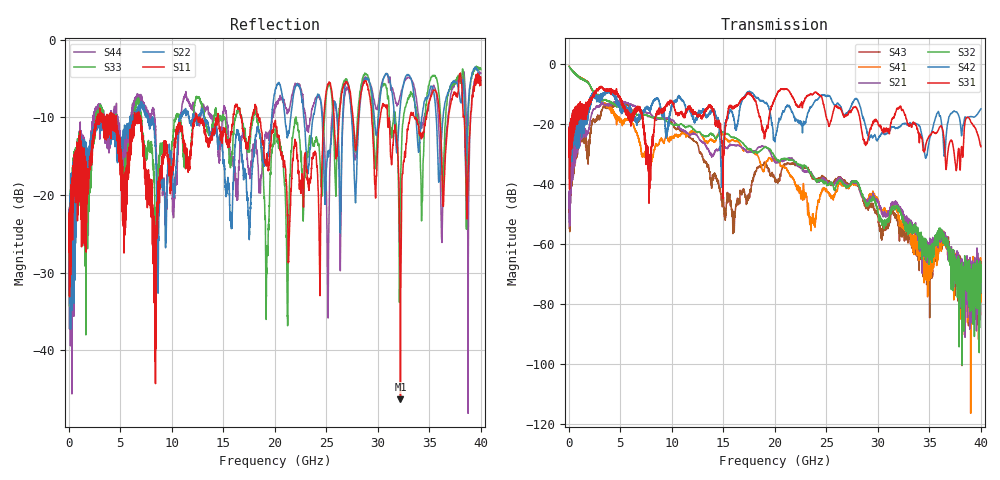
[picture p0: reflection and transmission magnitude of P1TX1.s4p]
!Agilent Technologies,N5245A,MY49151084,A.09.20.08
!Agilent N5245A: A.09.20.08
!Date: Thursday, March 01, 2012 10:29:25
!Correction: S11(Full 4 Port(1,2,3,4))
!S12(Full 4 Port(1,2,3,4))
!S13(Full 4 Port(1,2,3,4))
!S14(Full 4 Port(1,2,3,4))
!S21(Full 4 Port(1,2,3,4))
!S22(Full 4 Port(1,2,3,4))
!S23(Full 4 Port(1,2,3,4))
!S24(Full 4 Port(1,2,3,4))
!S31(Full 4 Port(1,2,3,4))
!S32(Full 4 Port(1,2,3,4))
!S33(Full 4 Port(1,2,3,4))
!S34(Full 4 Port(1,2,3,4))
!S41(Full 4 Port(1,2,3,4))
!S42(Full 4 Port(1,2,3,4))
!S43(Full 4 Port(1,2,3,4))
!S44(Full 4 Port(1,2,3,4))
!S4P File: Measurements: <S11,S12,S13,S14>,
!<S21,S22,S23,S24>,
!<S31,S32,S33,S34>,
!<S41,S42,S43,S44>:
# Hz S  dB  R 50
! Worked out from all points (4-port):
!   3996 points, 50 MHz to 40 GHz, reference 50 ohm
!   strongest paths, dB at 50 MHz, 10.04 GHz, 20.03 GHz, 30.02 GHz, 40 GHz:
!     S31: -23.6, -13.0, -11.5, -19.8, -27.5
!     S42: -23.5, -13.7, -25.9, -25.1, -15.0
!     S32: -0.8, -20.0, -31.2, -49.2, -67.6
!     S21: -43.5, -18.7, -32.8, -45.4, -76.0
!     S41: -0.7, -24.3, -31.7, -45.5, -64.7
!     S43: -44.3, -19.7, -38.9, -50.6, -71.4
!   lowest |S11| = -46.4 dB at 32.2 GHz (marker M1), VSWR 1.01, Z = 50.2 + j0.429 ohm
!   |S11| at or under -10 dB: start of sweep to 2.749 GHz; 6.99 GHz to 12.31 GHz (5.318 GHz wide, 55.1 % of centre); 18.41 GHz to 24.76 GHz (6.352 GHz wide, 29.4 % of centre)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
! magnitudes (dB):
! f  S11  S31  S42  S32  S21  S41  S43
! 50 MHz  -23.4  -23.6  -23.5  -0.8  -43.5  -0.7  -44.3
! 5.4 GHz  -22.8  -15.0  -13.9  -15.1  -12.7  -19.1  -13.0
! 7.79 GHz  -18.6  -38.8  -15.2  -17.3  -16.2  -36.9  -17.4
! 15.98 GHz  -9.7  -14.7  -17.6  -24.4  -26.9  -25.4  -49.6
! 21.75 GHz  -15.4  -11.2  -16.3  -32.0  -31.8  -38.1  -33.1
! 32.2 GHz  -46.4  -14.1  -20.9  -49.9  -48.1  -53.1  -54.5
! 40 GHz  -5.8  -27.5  -15.0  -67.6  -76.0  -64.7  -71.4
